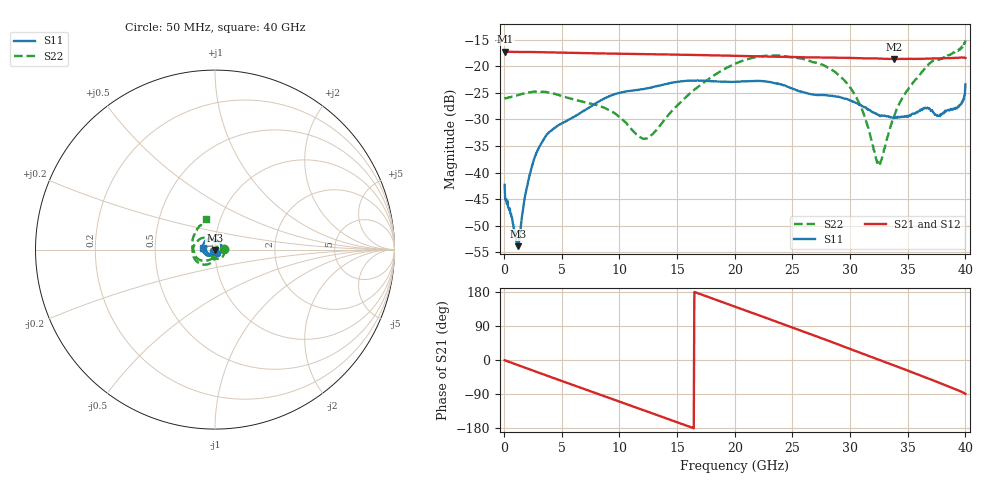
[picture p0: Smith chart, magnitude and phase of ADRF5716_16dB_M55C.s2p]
! Device: ADRF5716
! Description: 30GHz 2-Bit Digital Attenuator
! Frequency: 100 MHz – 30 GHz
! Ports:
! ATTIN  = Port 1
! ATTOUT = Port 2
! State: 16 dB Attenuation selected
! Supply Voltage:
! VDD  =  +3.30 Volts
! VSS  =  -3.30 Volts
! Control Voltages:
! D5 = 3.3V, D6 = 0V
! Temperature = -55 C
! Data: Data was collected using a calibrated network analyzer.
!  The reference plane is the package pins of ADRF5716 switch.
! Note: Analog Devices supplies this data as a sample of measured data for this product.
!  Your particular data for this product may vary.
!  Analog Devices reserves the right to change this data at anytime
# HZ S DB R 50
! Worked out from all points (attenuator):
!   800 points, 50 MHz to 40 GHz, reference 50 ohm
!   highest |S21| = -17.26 dB at 100 MHz (marker M1); lowest = -18.6 dB at 33.8 GHz (marker M2)
!   lowest |S11| = -53.9 dB at 1.2 GHz (marker M3), VSWR 1.00, Z = 49.9 - j0.14 ohm
!   |S11| at or under -10 dB: start of sweep to end of sweep
!   |S22| runs from -38.6 to -15.1 dB; largest |S21 - S12| = 0
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5e7  -42.30 -137.9  -17.26 -0.6  -17.26 -0.6  -26.11 2.4
1e8  -45.06 175.5  -17.26 -1.2  -17.26 -1.2  -25.99 -0.2
1.2e9  -53.85 -136.3  -17.30 -13.4  -17.30 -13.4  -25.43 -14.2
2.05e9  -42.10 -79.3  -17.31 -22.7  -17.31 -22.7  -24.97 -28.4
3e9  -35.39 -91.2  -17.32 -33.3  -17.32 -33.3  -24.77 -45.7
4e9  -32.24 -105.9  -17.37 -44.4  -17.37 -44.4  -25.00 -63.4
6.75e9  -28.59 -123.4  -17.51 -74.3  -17.51 -74.3  -26.62 -99.2
9.4e9  -25.40 -140.6  -17.61 -103.2  -17.61 -103.2  -28.58 -125.5
1.2e10  -24.29 -158.4  -17.69 -131.4  -17.69 -131.4  -33.56 -117.5
1.34e10  -23.63 -165.4  -17.74 -146.8  -17.74 -146.8  -31.49 -92.5
1.64e10  -22.68 173.8  -17.86 -179.4  -17.86 -179.4  -24.59 -96.8
2.005e10  -22.90 151.3  -18.02 140.4  -18.02 140.4  -19.49 -128.1
2.67e10  -25.27 95.4  -18.33 66.8  -18.33 66.8  -19.16 156.9
3.015e10  -26.55 50.7  -18.43 27.5  -18.43 27.5  -24.43 105.0
3.12e10  -27.64 32.7  -18.50 15.3  -18.50 15.3  -29.04 79.4
3.245e10  -29.15 13.6  -18.54 1.1  -18.54 1.1  -38.33 -2.5
3.335e10  -29.45 0.7  -18.60 -9.1  -18.60 -9.1  -32.40 -71.1
3.38e10  -29.73 -5.5  -18.64 -14.2  -18.64 -14.2  -29.51 -87.5
3.675e10  -27.82 -70.8  -18.55 -48.5  -18.55 -48.5  -19.79 -146.0
3.76e10  -29.37 -90.1  -18.49 -58.6  -18.49 -58.6  -18.79 -167.3
3.925e10  -27.93 -135.0  -18.40 -78.6  -18.40 -78.6  -17.17 150.5
4e10  -23.40 173.5  -18.43 -89.2  -18.43 -89.2  -15.13 105.7
